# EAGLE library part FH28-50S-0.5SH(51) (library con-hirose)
Flexible Printed Circuit & Flexible Flat Cable ZIF Connectors 0.5 mm Pitch, 2.55 mm above the board Source: http://www.hirose.co.jp/cataloge_hp/e58618038.pdf
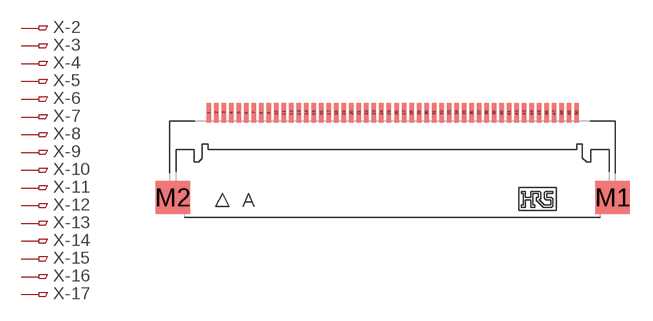
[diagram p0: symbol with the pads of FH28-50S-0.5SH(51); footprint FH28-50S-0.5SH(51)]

Designator prefix X; gates -2=PIN -3=PIN -4=PIN -5=PIN -6=PIN -7=PIN -8=PIN -9=PIN -10=PIN -11=PIN -12=PIN -13=PIN -14=PIN -15=PIN -16=PIN -17=PIN -18=PIN -19=PIN -20=PIN -21=PIN -22=PIN -23=PIN -24=PIN -25=PIN -26=PIN -27=PIN -28=PIN -29=PIN -30=PIN -31=PIN -32=PIN -33=PIN -34=PIN -35=PIN -36=PIN -37=PIN -38=PIN -39=PIN -40=PIN -41=PIN -42=PIN -43=PIN -44=PIN -45=PIN -46=PIN -47=PIN -48=PIN -49=PIN -50=PIN -1=PINV

## FH28-50S-0.5SH(51) (OC_FARNELL: unknown; OC_NEWARK: unknown)  [FH28-50S-0.5SH(51)]
1  -1:1  pas
2  -2:1  pas
3  -3:1  pas
4  -4:1  pas
5  -5:1  pas
6  -6:1  pas
7  -7:1  pas
8  -8:1  pas
9  -9:1  pas
10  -10:1  pas
11  -11:1  pas
12  -12:1  pas
13  -13:1  pas
14  -14:1  pas
15  -15:1  pas
16  -16:1  pas
17  -17:1  pas
18  -18:1  pas
19  -19:1  pas
20  -20:1  pas
21  -21:1  pas
22  -22:1  pas
23  -23:1  pas
24  -24:1  pas
25  -25:1  pas
26  -26:1  pas
27  -27:1  pas
28  -28:1  pas
29  -29:1  pas
30  -30:1  pas
31  -31:1  pas
32  -32:1  pas
33  -33:1  pas
34  -34:1  pas
35  -35:1  pas
36  -36:1  pas
37  -37:1  pas
38  -38:1  pas
39  -39:1  pas
40  -40:1  pas
41  -41:1  pas
42  -42:1  pas
43  -43:1  pas
44  -44:1  pas
45  -45:1  pas
46  -46:1  pas
47  -47:1  pas
48  -48:1  pas
49  -49:1  pas
50  -50:1  pas

## Footprint FH28-50S-0.5SH(51) (pad centres in mm)
Flexible Printed Circuit & Flexible Flat Cable ZIF Connectors 0.5 mm Pitch, 2.55 mm above the board Source: http://www.hirose.co.jp/cataloge_hp/e58618038.pdf
smd 0.3 x 1.3: 1 -12.25,3.5; 2 -11.75,3.5; 3 -11.25,3.5; 4 -10.75,3.5; 5 -10.25,3.5; 6 -9.75,3.5; 7 -9.25,3.5; 8 -8.75,3.5; 9 -8.25,3.5; 10 -7.75,3.5; 11 -7.25,3.5; 12 -6.75,3.5; 13 -6.25,3.5; 14 -5.75,3.5; 15 -5.25,3.5; 16 -4.75,3.5; 17 -4.25,3.5; 18 -3.75,3.5; 19 -3.25,3.5; 20 -2.75,3.5; 21 -2.25,3.5; 22 -1.75,3.5; 23 -1.25,3.5; 24 -0.75,3.5; 25 -0.25,3.5; 26 0.25,3.5; 27 0.75,3.5; 28 1.25,3.5; 29 1.75,3.5; 30 2.25,3.5; 31 2.75,3.5; 32 3.25,3.5; 33 3.75,3.5; 34 4.25,3.5; 35 4.75,3.5; 36 5.25,3.5; 37 5.75,3.5; 38 6.25,3.5; 39 6.75,3.5; 40 7.25,3.5; 41 7.75,3.5; 42 8.25,3.5; 43 8.75,3.5; 44 9.25,3.5; 45 9.75,3.5; 46 10.25,3.5; 47 10.75,3.5; 48 11.25,3.5; 49 11.75,3.5; 50 12.25,3.5
smd 2.3 x 2.2: M1 14.65,-2.15; M2 -14.65,-2.15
